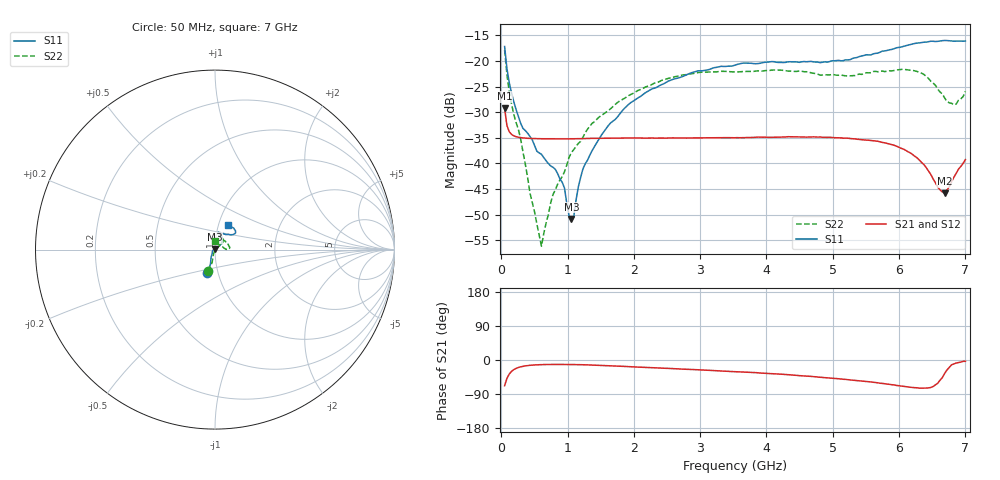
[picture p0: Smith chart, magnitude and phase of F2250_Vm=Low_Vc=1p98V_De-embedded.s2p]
! Integrated Device Technology
! Corporate Headquarters
! 6024 Silver Creek Valley Road
! San Jose, CA 95138  USA
! Phone:  1-408-284-8200
! Toll Free:  1-800-223-1366
! Webpage:  http://www.idt.com/
! Timing and RF Division
! 515 Groton Road, Suite 102
! Westford, MA 01886-6024
! Device:  F2250
! Description: Voltage Variable RF Attenuator
! Frequency:  50.0 -  6000.00 MHz
! Package:  3x3 mm Thin QFN Plastic Package: 16 pin
! Ports:  2 RF, 3 DC
!  Pin  1  = GND
!  Pin  2  = NC
!  Pin  3  = RF1  = Port 1
!  Pin  4  = NC
!  Pin  5  = GND
!  Pin  6  = GND
!  Pin  7  = GND
!  Pin  8  = GND
!  Pin  9  = NC
!  Pin 10  = RF2  = Port 2
!  Pin 11  = NC
!  Pin 12  = GND
!  Pin 13  = GND
!  Pin 14  = VCNTRL
!  Pin 15  = VDD
!  Pin 16  = VMODE
! Vcntrl:  1.980 Volts
! Vmode:  +0.000 Volts
! Vdd:  +3.30  Volts
! Current:  1.181 mA
! Data:  The device was measured on a the F2250 evaluation board which has
!  individual transmission lines to the RF pins.  Data was collected
!  using a calibrated network analyzer.  The evaluation board was
!  de-embedded using a TRL calibration technique.
!  The reference plane is the edge of the package pin.
! Misc:  SN 10
!  Action Tracker AT0258
! Date Measured:  2014-11-26
! Date:  2015-10-15  MJV
! Note:
!  Integrated Device Technology supplies this data as a sample of measured
!  data at the package pin for this product.  Your particular data for this
!  product may vary.
!  Data was taken at 25 degrees C.
!  Integrated Device Technology reserves the right to change this data at anytime.
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# GHz S dB R 50
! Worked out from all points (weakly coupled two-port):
!   201 points, 50 MHz to 7 GHz, reference 50 ohm
!   highest |S21| = -29.24 dB at 50 MHz (marker M1); lowest = -45.8 dB at 6.687 GHz (marker M2)
!   lowest |S11| = -50.8 dB at 1.058 GHz (marker M3), VSWR 1.01, Z = 49.8 + j0.243 ohm
!   |S11| at or under -10 dB: start of sweep to end of sweep
!   |S22| runs from -56.2 to -17.9 dB; largest |S21 - S12| = 5.7e-05
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0.05  -17.18 -108.6  -29.24 -68.0  -29.24 -67.9  -17.89 -107.9
0.08475  -21.44 -107.4  -32.60 -48.7  -32.60 -48.7  -22.61 -102.6
0.1195  -24.20 -111.7  -33.80 -37.2  -33.79 -37.2  -25.95 -104.5
0.29325  -32.20 -127.5  -34.97 -18.0  -34.97 -17.9  -35.28 -106.5
0.43225  -34.76 -144.5  -35.12 -14.0  -35.12 -14.0  -45.78 -124.0
0.606  -38.21 -160.7  -35.19 -12.2  -35.18 -12.2  -56.16 137.9
0.77975  -40.75 177.6  -35.22 -11.7  -35.21 -11.7  -46.08 72.5
0.91875  -43.68 158.0  -35.21 -11.7  -35.21 -11.7  -42.58 58.5
1.023  -50.24 143.7  -35.21 -11.9  -35.20 -11.9  -38.80 56.4
1.05775  -50.83 122.1  -35.20 -11.9  -35.20 -11.9  -37.87 54.7
1.0925  -50.41 88.6  -35.19 -12.0  -35.19 -12.0  -37.31 51.4
1.162  -44.58 56.3  -35.18 -12.2  -35.17 -12.2  -36.09 44.8
1.2315  -41.07 43.6  -35.15 -12.5  -35.15 -12.5  -34.92 40.3
1.6485  -32.10 41.8  -35.07 -15.2  -35.07 -15.2  -29.33 41.9
2.37825  -24.87 47.3  -35.04 -21.1  -35.05 -21.1  -24.07 44.9
3.525  -20.81 72.4  -34.99 -30.7  -35.00 -30.7  -22.16 68.3
4.7065  -20.17 72.3  -34.82 -43.9  -34.82 -43.9  -22.40 68.5
5.85325  -17.82 40.4  -36.21 -64.3  -36.21 -64.3  -21.92 16.4
6.33975  -16.40 40.9  -39.82 -74.3  -39.83 -74.2  -22.39 2.2
6.68725  -15.99 48.8  -45.83 -35.3  -45.80 -35.0  -27.21 22.6
6.861  -16.12 55.1  -41.94 -8.0  -41.91 -7.9  -28.41 58.8
7  -16.12 63.2  -39.25 -3.4  -39.21 -3.6  -25.93 88.1
